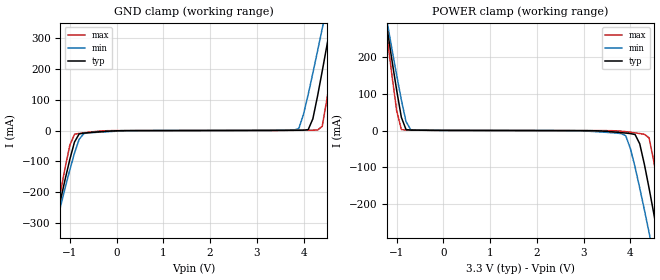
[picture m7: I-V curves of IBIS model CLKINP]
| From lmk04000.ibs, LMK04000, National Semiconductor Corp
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|   Model CLKINP
[Model]  CLKINP
Model_type Input
Polarity   Non-Inverting
Vinl =   -150m
Vinh =   +150m
C_comp   1.0200pF   NA   NA
[Temperature Range]   25.0000   85.0000   -40.0000
[Voltage Range]   3.3000V   3.1500V   3.4500V
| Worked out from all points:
|   GND clamp passes 1 mA (typ) near -0.02 V on its own axis
|   POWER clamp passes 1 mA (typ) near -0.59 V on its own axis
[GND_clamp]
|Voltage   I(typ)   I(min)   I(max)
-3.3V     -1.732A    -1.58A     -1.981A
-1.4V     -367.6mA   -371.9mA   -366.7mA
-900mV    -37.4mA    -73.16mA   -12.14mA
-600mV    -7.015mA   -7.508mA   -5.506mA
3.9V      1.018mA    6.73mA     749.5uA
4.1V      2.747mA    116.4mA    1.044mA
4.3V      111.1mA    257mA      1.47mA
4.4V      191.7mA    329.3mA    13.5mA
4.6V      358.6mA    475.3mA    199.9mA
4.7V      443mA      548.7mA    302.2mA
4.8V      527.8mA    622.3mA    405.6mA
6.5V      1.973A     1.876A     2.172A
[POWER_clamp]
|Voltage   I(typ)   I(min)   I(max)
-3.3V     2.066A     1.839A     2.275A
-1.3V     358.3mA    365.7mA    353.8mA
-1.2V     273.9mA    293.1mA    250.9mA
-900mV    36.15mA    83.39mA    2.654mA
-700mV    1.182mA    2.416mA    1.121mA
3.8V      -5.664mA   -8.223mA   -1.786mA
4.1V      -10.85mA   -99.61mA   -6.395mA
4.3V      -92.42mA   -216.5mA   -10.3mA
4.4V      -157.1mA   -278.1mA   -19.98mA
4.6V      -296.1mA   -403.3mA   -160mA
4.8V      -439.2mA   -529.7mA   -324.5mA
6.5V      -1.666A    -1.58A     -1.77A
